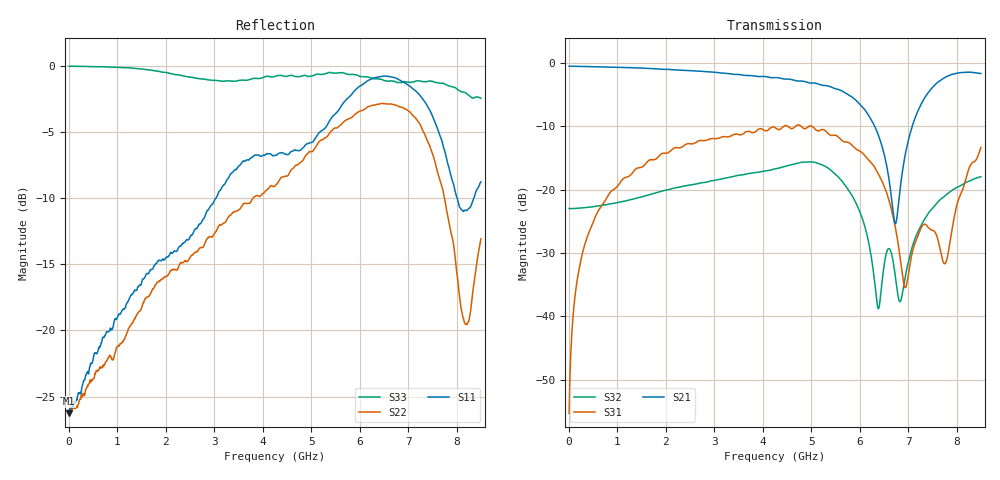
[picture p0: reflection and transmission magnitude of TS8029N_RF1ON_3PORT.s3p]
!Created with skrf (http://scikit-rf.org).
# GHz S RI R 50.0
!freq ReS11 ImS11 ReS12 ImS12 ReS13 ImS13
! ReS21 ImS21 ReS22 ImS22 ReS23 ImS23
! ReS31 ImS31 ReS32 ImS32 ReS33 ImS33
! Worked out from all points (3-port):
!   1601 points, 10 MHz to 8.5 GHz, reference 50 ohm
!   strongest paths, dB at 10 MHz, 2.132 GHz, 4.255 GHz, 6.378 GHz, 8.5 GHz:
!     S21: -0.5, -1.0, -2.3, -11.2, -1.6
!     S31: -55.3, -13.7, -10.2, -17.3, -13.3
!     S32: -23.0, -19.8, -16.7, -38.7, -18.0
!   lowest |S11| = -26.3 dB at 10 MHz (marker M1), VSWR 1.10, Z = 55.1 - j0.101 ohm
!   |S11| at or under -10 dB: start of sweep to 3.038 GHz; 8.011 GHz to 8.357 GHz (346.4 MHz wide, 4.23 % of centre)
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0.01  0.0486 -0.000912  0.9457 -0.00493  0.000707 0.00156
      0.9458 -0.00503  0.0496 -0.00213  0.071 -1.67e-05
      0.000726 0.00155  0.071 3.08e-05  0.9952 -0.00813
0.2381688  0.0458 -0.035  0.9369 -0.0907  0.00411 0.0258
           0.9373 -0.0905  0.0464 -0.0297  0.0716 0.000785
           0.00412 0.0258  0.0716 0.000723  0.9808 -0.1631
0.8536938  0.0172 -0.0994  0.8769 -0.3066  0.0448 0.0837
           0.8768 -0.3067  0.0173 -0.0782  0.0771 -0.000765
           0.0449 0.0838  0.0772 -0.000717  0.8306 -0.5358
4.255  -0.4398 -0.1286  -0.0877 -0.7635  0.2116 -0.2265
       -0.0883 -0.7628  -0.3183 0.148  0.0687 -0.1285
       0.2107 -0.2266  0.0685 -0.1288  -0.8005 -0.4346
6.0379  -0.6675 0.5162  -0.3967 -0.2305  -0.095 -0.1737
        -0.397 -0.2306  0.0369 0.6757  -0.0562 -0.0259
        -0.0948 -0.1738  -0.0562 -0.0259  -0.64 0.6462
6.3775  -0.5699 0.7045  -0.2638 -0.0813  -0.107 -0.0834
        -0.2637 -0.081  0.2652 0.6642  -0.00627 -0.00982
        -0.107 -0.0835  -0.00629 -0.0098  -0.3721 0.81
6.664038  -0.406 0.8096  -0.0711 -0.0398  -0.0641 -0.0216
          -0.0712 -0.0398  0.5159 0.4956  -0.00942 -0.0288
          -0.0641 -0.0214  -0.00942 -0.0289  0.0318 0.876
6.934656  -0.1624 0.8452  0.1191 -0.1405  -0.00816 -0.0148
          0.1192 -0.1405  0.6623 0.1794  0.0146 -0.0134
          -0.0081 -0.0148  0.0146 -0.0135  0.4258 0.7603
7.725288  0.3104 0.3873  -0.1022 -0.7477  -0.0263 0.00518
          -0.1024 -0.7493  0.1715 -0.2869  0.0447 -0.075
          -0.0262 0.00516  0.0446 -0.075  0.8533 0.0898
8.5  -0.0753 0.3561  -0.6276 -0.538  0.2124 0.0331
     -0.6288 -0.5373  -0.1898 0.1145  0.0312 -0.1227
     0.2129 0.0325  0.0312 -0.1227  0.0184 -0.7529
